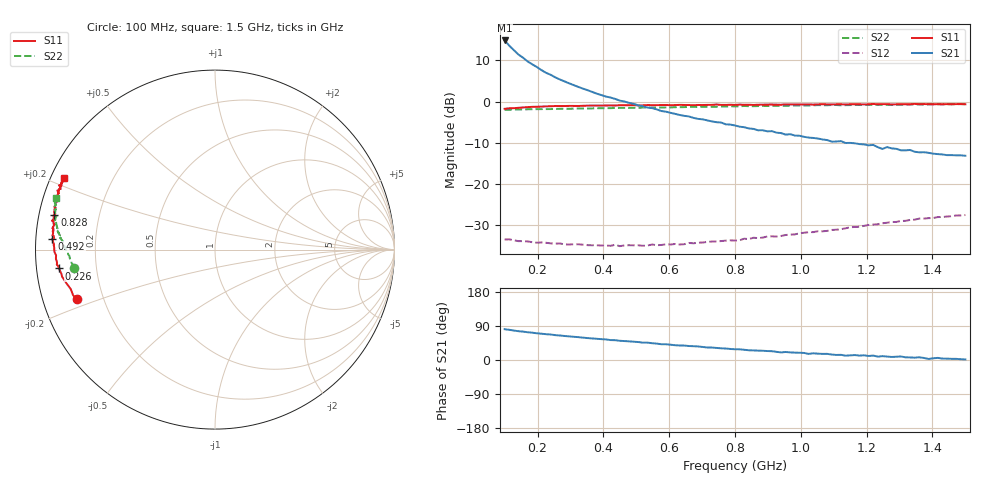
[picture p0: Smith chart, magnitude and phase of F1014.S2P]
!  POLYFET RF DEVICES
!  F1014
!  S PARAMETERS
!  VDS=28V, IDQ=400mA
! Date: Mon Oct 21 17:59:02 1991
! Bias (V mA) : V1=2.0480000  I1=0.0039989  V2=27.998000  I2=408.05560
# MHZ S MA R 50
!  FREQ  S11 MAG  S11 ANG  S21 MAG  S21 ANG  S12 MAG  S12 ANG  S22 MAG  S22 ANG
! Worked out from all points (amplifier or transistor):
!   101 points, 100 MHz to 1.5 GHz, reference 50 ohm
!   highest |S21| = 14.9 dB at 100 MHz (marker M1)
!   |S21| within 3 dB of that: start of sweep to 136.6 MHz
!   unconditionally stable (mu >= 1): 352.7 MHz to end of sweep
!   at 324 MHz: K = 0.94, MSG = 19.1 dB, |S12| = -34.6 dB
!   at 800 MHz: K = 1.77, MAG = 8.9 dB, |S12| = -33.7 dB
!   at 1.5 GHz: K = 1.12, MAG = 5.1 dB, |S12| = -27.5 dB
!   S11 on the Smith chart (normalised r, x): 100 MHz: 0.10, -0.17; 226 MHz: 0.07, -0.06; 492 MHz: 0.05, +0.03; 828 MHz: 0.04, +0.11; 1.5 GHz: 0.04, +0.22
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100  0.8182 -160.4  5.527 81.3  0.02123 2.0  0.7951 -172.4
114  0.8302 -162.1  4.786 79.7  0.02131 0.5  0.7961 -173.0
128  0.8332 -164.6  4.22 77.7  0.0208 1.8  0.7992 -174.3
142  0.8415 -166.1  3.731 76.0  0.02026 1.8  0.8029 -174.7
170  0.8575 -168.8  3.071 73.2  0.02011 1.4  0.8074 -175.8
212  0.8702 -171.9  2.414 69.4  0.01957 2.6  0.8114 -177.1
226  0.8761 -173.1  2.237 68.1  0.01936 4.1  0.8118 -177.3
268  0.8834 -175.1  1.857 64.7  0.01899 6.0  0.818 -178.1
296  0.8877 -176.6  1.668 62.3  0.01844 6.1  0.8194 -178.8
338  0.8905 -178.6  1.439 59.0  0.01835 8.6  0.8246 -179.3
408  0.8977 178.6  1.152 54.2  0.01793 13.4  0.8336 179.7
450  0.9042 177.3  1.029 50.7  0.01761 16.2  0.8388 178.9
492  0.9088 176.1  0.941 48.3  0.01804 19.4  0.8438 178.3
576  0.9091 173.8  0.7693 41.6  0.0182 25.6  0.8497 177.1
716  0.9128 170.4  0.5921 33.0  0.01983 33.8  0.8695 175.0
800  0.9123 168.6  0.5133 28.3  0.02061 38.4  0.8758 173.8
828  0.9148 167.9  0.4893 27.0  0.02171 39.9  0.8858 173.0
1038  0.9198 163.2  0.3624 17.7  0.02607 48.5  0.9024 169.9
1220  0.9377 159.4  0.2984 11.7  0.03216 53.5  0.918 166.7
1248  0.9328 158.8  0.2665 10.1  0.03341 54.9  0.9166 166.1
1276  0.9233 158.5  0.2708 8.1  0.03464 54.5  0.9166 165.9
1500  0.9288 154.6  0.2203 1.5  0.04208 53.8  0.9312 162.1
